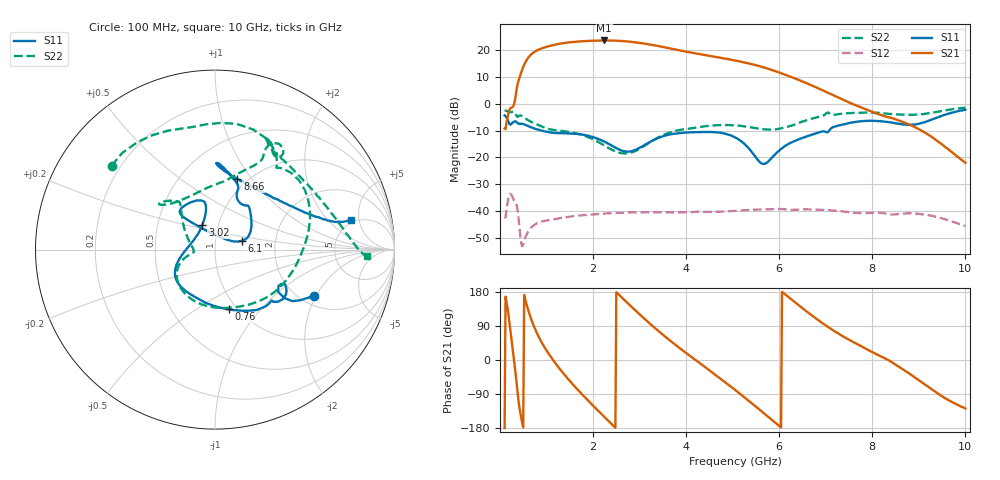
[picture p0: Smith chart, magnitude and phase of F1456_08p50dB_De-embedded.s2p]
! Integrated Device Technology
! Corporate Headquarters
! 6024 Silver Creek Valley Road
! San Jose, CA 95138  USA
! Phone:  1-408-284-8200
! Toll Free:  1-800-223-1366
! Webpage:  http://www.idt.com/
! Timing and RF Division
! 515 Groton Road, Suite 102
! Westford, MA 01886-6024
! Device:  F1456
! Description: 6-bit 0.5 dB Transmit Variable Gain Amplifier
! Frequency:  2100.0 -  2950.00 MHz
! Package:  6x6 mm Thin QFN Plastic Package: 28 pin
! State:  17
! Atten State:  8.5 dB
! Voltage:  +5.00 Volts
! Current:  217.026 mA
! Data:  The device was measured on a the F1455 evaluation board which has
!  individual transmission lines to the RF pins.  Data was collected
!  using a calibrated network analyzer.  The evaluation board was
!  de-embedded using a TRL calibration technique.
!  The reference plane is the edge of the package pin.
!  Pin  1 = CSb
!  Pin  2 = DATA
!  Pin  3 = CLK
!  Pin  4 = RSET
!  Pin  5 = GND
!  Pin  6 = RFIN  = Port 1
!  Pin  7 = GND
!  Pin  8 = NC
!  Pin  9 = NC
!  Pin 10 = NC
!  Pin 11 = NC
!  Pin 12 = NC
!  Pin 13 = NC
!  Pin 14 = /STBY
!  Pin 15 = GND
!  Pin 16 = RFOUT  = Port 2
!  Pin 17 = GND
!  Pin 18 = NC
!  Pin 19 = NC
!  Pin 20 = NC
!  Pin 21 = GND
!  Pin 22 = NC
!  Pin 23 = GND
!  Pin 24 = NC
!  Pin 25 = NC
!  Pin 26 = NC
!  Pin 27 = GND
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# GHz S dB R 50
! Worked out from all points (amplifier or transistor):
!   496 points, 100 MHz to 10 GHz, reference 50 ohm
!   highest |S21| = 23.7 dB at 2.24 GHz (marker M1)
!   |S21| within 3 dB of that: 892.6 MHz to 3.664 GHz (2.771 GHz wide, 122 % of centre)
!   unconditionally stable (mu >= 1): start of sweep to end of sweep
!   at 1.74 GHz: K = 3.68, MAG = 23.9 dB, |S12| = -41.7 dB
!   at 5.06 GHz: K = 6.29, MAG = 17.1 dB, |S12| = -40.0 dB
!   at 10 GHz: K = 138.52, MAG = -12.7 dB, |S12| = -45.6 dB
!   S11 on the Smith chart (normalised r, x): 100 MHz: 2.33, -1.92; 760 MHz: 0.92, -0.69; 3.02 GHz: 0.84, +0.23; 6.1 GHz: 1.34, +0.14; 8.66 GHz: 0.90, +0.85; 10 GHz: 4.58, +3.81
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0.1  -4.33 -25.3  -9.25 -179.5  -42.34 45.2  -2.60 141.0
0.32  -6.59 -32.4  1.12 -18.5  -36.62 -136.2  -3.35 64.5
0.44  -7.43 -44.3  10.87 -141.6  -49.75 143.3  -4.34 39.5
0.58  -8.09 -59.6  16.54 143.1  -48.56 177.6  -5.88 5.3
0.76  -9.37 -77.1  19.64 80.1  -45.01 133.0  -7.44 -26.7
0.98  -10.35 -98.1  21.19 29.0  -43.70 92.0  -9.08 -62.8
1.2  -10.90 -115.7  22.18 -9.9  -43.03 66.5  -9.86 -92.3
1.5  -11.07 -134.0  22.99 -55.2  -42.17 40.3  -10.56 -124.5
1.76  -11.47 -146.2  23.37 -90.1  -41.67 22.1  -11.62 -144.0
2.24  -14.12 -167.7  23.68 -149.8  -41.01 -6.5  -15.53 -165.7
2.6  -17.35 163.5  23.50 167.0  -40.73 -26.0  -18.43 -173.5
3.02  -16.27 117.4  22.73 118.3  -40.55 -47.7  -16.53 163.3
3.4  -12.79 102.7  21.60 77.0  -40.59 -65.9  -12.59 139.4
4.1  -10.64 113.2  19.17 9.5  -40.48 -95.1  -9.18 128.9
4.6  -10.58 130.3  17.65 -36.5  -40.37 -116.6  -8.07 137.7
5.06  -12.61 133.4  16.16 -79.7  -40.00 -136.1  -8.05 140.7
5.6  -22.03 85.1  13.96 -133.3  -39.49 -163.8  -9.39 127.3
6.1  -16.07 18.2  11.03 175.8  -39.37 166.6  -8.91 91.6
6.7  -11.55 40.3  6.86 117.7  -39.49 133.0  -5.55 64.4
8.36  -6.87 85.5  -5.06 -1.3  -41.34 60.4  -3.77 62.3
8.66  -7.69 72.4  -6.82 -24.7  -41.02 52.0  -4.04 53.1
10  -2.23 12.5  -22.07 -127.9  -45.57 -27.3  -1.46 -2.5
